(* Logix 5000 Controller export DH485RouterExample; controller DH485RouterExample 1756-L62 rev 19.11; software revision 19.01 *)

TASK MainTask (continuous, watchdog 500 ms) : MainProgram

MODULES
   Local : 1756-L62 (ICP 0, rev 19.11)
      Ethernet : 1756-EN2TR (ICP 1, Ethernet 192.168.1.101, rev 3.1)
         DH485R01 : ETHERNET-MODULE (Ethernet 192.168.1.41, rev 1.1, Output RPI 500 ms)
END_MODULES

TYPE AparianDH485RDH485Status :
STRUCT
   TransparentPCCCMode : BOOL;
   ReactiveTagMode : BOOL;
   ScheduledTagMode : BOOL;
   UnscheduledMode : BOOL;
   ConfigurationValid : BOOL;
   RoutingInhibited : BOOL;
   Reserved1 : BOOL;
   Reserved2 : BOOL;
   ScheduledTagStatus0 : BOOL;
   ScheduledTagStatus1 : BOOL;
   ScheduledTagStatus2 : BOOL;
   ScheduledTagStatus3 : BOOL;
   ScheduledTagStatus4 : BOOL;
   ScheduledTagStatus5 : BOOL;
   ScheduledTagStatus6 : BOOL;
   ScheduledTagStatus7 : BOOL;
   ScheduledTagStatus8 : BOOL;
   ScheduledTagStatus9 : BOOL;
   ScheduledTagStatus10 : BOOL;
   ScheduledTagStatus11 : BOOL;
   ScheduledTagStatus12 : BOOL;
   ScheduledTagStatus13 : BOOL;
   ScheduledTagStatus14 : BOOL;
   ScheduledTagStatus15 : BOOL;
   ScheduledTagStatus16 : BOOL;
   ScheduledTagStatus17 : BOOL;
   ScheduledTagStatus18 : BOOL;
   ScheduledTagStatus19 : BOOL;
END_STRUCT
END_TYPE

TYPE AparianDH485RInput :
STRUCT
   Instance : STRING;
   Status : AparianDH485RDH485Status;
   TransactionRate : DINT;
   Temperature : REAL;
   DH485RxPacketCount : DINT;
   DH485TxPacketCount : DINT;
   DH485ChecksumErrors : DINT;
   PCCCRequests : DINT;
   PCCCFailures : DINT;
   TagReads : DINT;
   TagWrites : DINT;
   TagConnectionFailures : DINT;
   TagErrors : DINT;
END_STRUCT
END_TYPE

TYPE AparianDH485RMsgDataType :
STRUCT
   BOOLEAN : BOOL;
   INT : BOOL;
   REAL : BOOL;
END_STRUCT
END_TYPE

TYPE AparianDH485RMsgFunctionType :
STRUCT
   PLC5TypedRead : BOOL;
   PLC5TypedWrite : BOOL;
   SLCTypedRead : BOOL;
   SLCTypedWrite : BOOL;
END_STRUCT
END_TYPE

TYPE AparianDH485RMsgRequest :
STRUCT
   DestinationNode : SINT;
   DF1DataFileAddress : STRING;
   Function : AparianDH485RMsgFunctionType;
   DataType : AparianDH485RMsgDataType;
   ElementCount : INT;
   RequestData : INT[128];
END_STRUCT
END_TYPE

TYPE AparianDH485RMsgResponse :
STRUCT
   Status : INT;
   ResponseLength : INT;
   ResponseData : INT[128];
END_STRUCT
END_TYPE

TYPE AparianDH485ROutput :
STRUCT
   RoutingInhibit : BOOL;
END_STRUCT
END_TYPE

VAR_GLOBAL   (* controller tags *)
   DH485R01Input : AparianDH485RInput := (Instance := 'South', Status.ReactiveTagMode := 1, Status.ConfigurationValid := 1, TransactionRate := 31, Temperature := 46.3, DH485RxPacketCount := 34218, DH485TxPacketCount := 34217, TagReads := 16522, TagWrites := 587);
   DH485R01Output : AparianDH485ROutput;
   DH485RMessage : MESSAGE;
        MessageParameters(MessageType := CIP Generic, RequestedLength := 360, ConnectedFlag := 2, ConnectionPath := DH485R01, ServiceCode := 16#006a, ObjectType := 16#0408, TargetObject := 1, LocalElement := DH485RMsgRequest, DestinationTag := DH485RMsgeResponse)
   DH485RMsgeResponse : AparianDH485RMsgResponse;
   DH485RMsgRequest : AparianDH485RMsgRequest := (DestinationNode := 5, DF1DataFileAddress := 'N10:0', Function.PLC5TypedRead := 1, DataType.INT := 1, ElementCount := 16);
   DH485RMsgTrigger : BOOL;
END_VAR

PROGRAM MainProgram   (* main routine MainRoutine *)

ROUTINE DH485Router   (* ladder *)
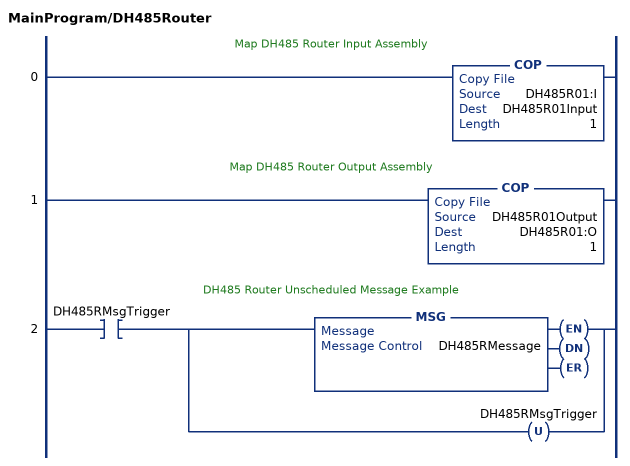
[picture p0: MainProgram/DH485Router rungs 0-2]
   // Map DH485 Router Input Assembly
   0: COP(DH485R01:I,DH485R01Input,1);
   // Map DH485 Router Output Assembly
   1: COP(DH485R01Output,DH485R01:O,1);
   // DH485 Router Unscheduled Message Example
   2: XIC(DH485RMsgTrigger)[MSG(DH485RMessage) ,OTU(DH485RMsgTrigger) ];
END_ROUTINE

ROUTINE MainRoutine   (* ladder *)
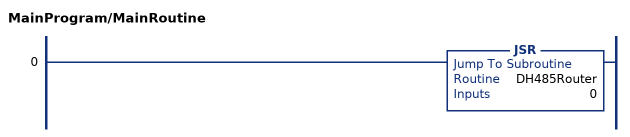
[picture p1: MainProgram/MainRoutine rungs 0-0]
   0: JSR(DH485Router,0);
END_ROUTINE
END_PROGRAM
